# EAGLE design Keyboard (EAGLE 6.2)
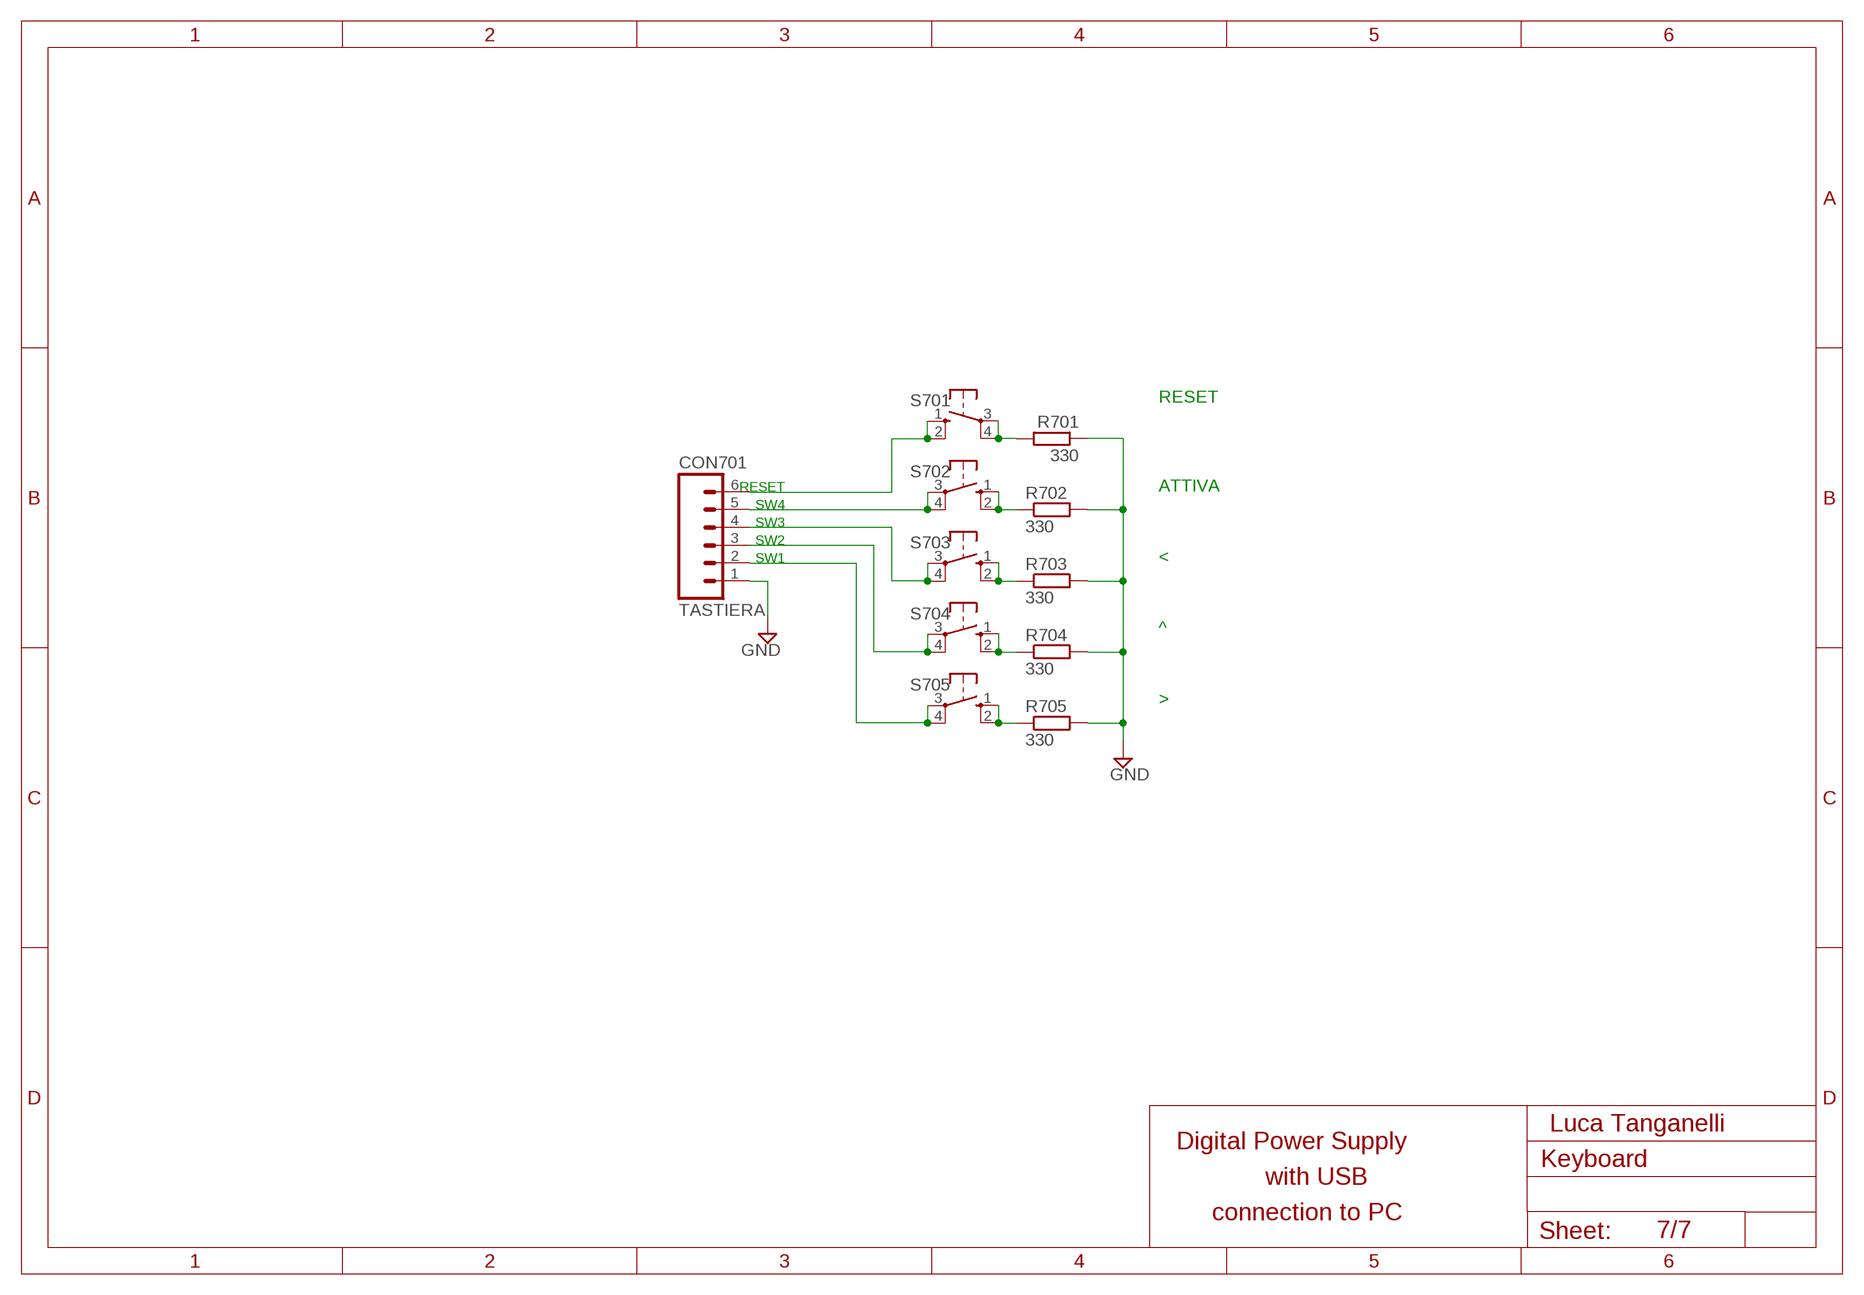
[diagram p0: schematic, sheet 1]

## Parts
CON701  TASTIERA  MA06  [06PA]
R701  330  R-EU_0207/10  [0207/10]
R702  330  R-EU_0207/10  [0207/10]
R703  330  R-EU_0207/10  [0207/10]
R704  330  R-EU_0207/10  [0207/10]
R705  330  R-EU_0207/10  [0207/10]
S701  10-XX  [B3F-10XX]
S702  10-XX  [B3F-10XX]
S703  10-XX  [B3F-10XX]
S704  10-XX  [B3F-10XX]
S705  10-XX  [B3F-10XX]

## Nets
GND: CON701.1 R701.1 R702.2 R703.2 R704.2 R705.2
N$1: CON701.5 S702.3(P) S702.4(P1)
N$2: CON701.4 S703.3(P) S703.4(P1)
N$3: CON701.3 S704.3(P) S704.4(P1)
N$4: CON701.2 S705.3(P) S705.4(P1)
N$10: R705.1 S705.1(S) S705.2(S1)
N$32: R701.2 S701.3(P) S701.4(P1)
N$86: R704.1 S704.1(S) S704.2(S1)
N$87: R703.1 S703.1(S) S703.2(S1)
N$88: R702.1 S702.1(S) S702.2(S1)
RESET1: CON701.6 S701.1(S) S701.2(S1)

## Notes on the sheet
- RESET
- RESET | ATTIVA
- SW4
- SW3
- SW2
- SW1 | <
- ^
- >
- Luca Tanganelli
- Digital Power Supply
- with USB
- connection to PC
- 7/7

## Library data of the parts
CON701 = #-con-amp-quick:MA06: AMP QUICK CONNECTOR; OC_FARNELL: unknown; OC_NEWARK: unknown
R701-R705 = #-rcl:R-EU_: RESISTOR, European symbol
S701-S705 = #-switch-omron:10-XX: OMRON SWITCH; MPN: B3F-1000; OC_FARNELL: 176432; OC_NEWARK: 36M3542

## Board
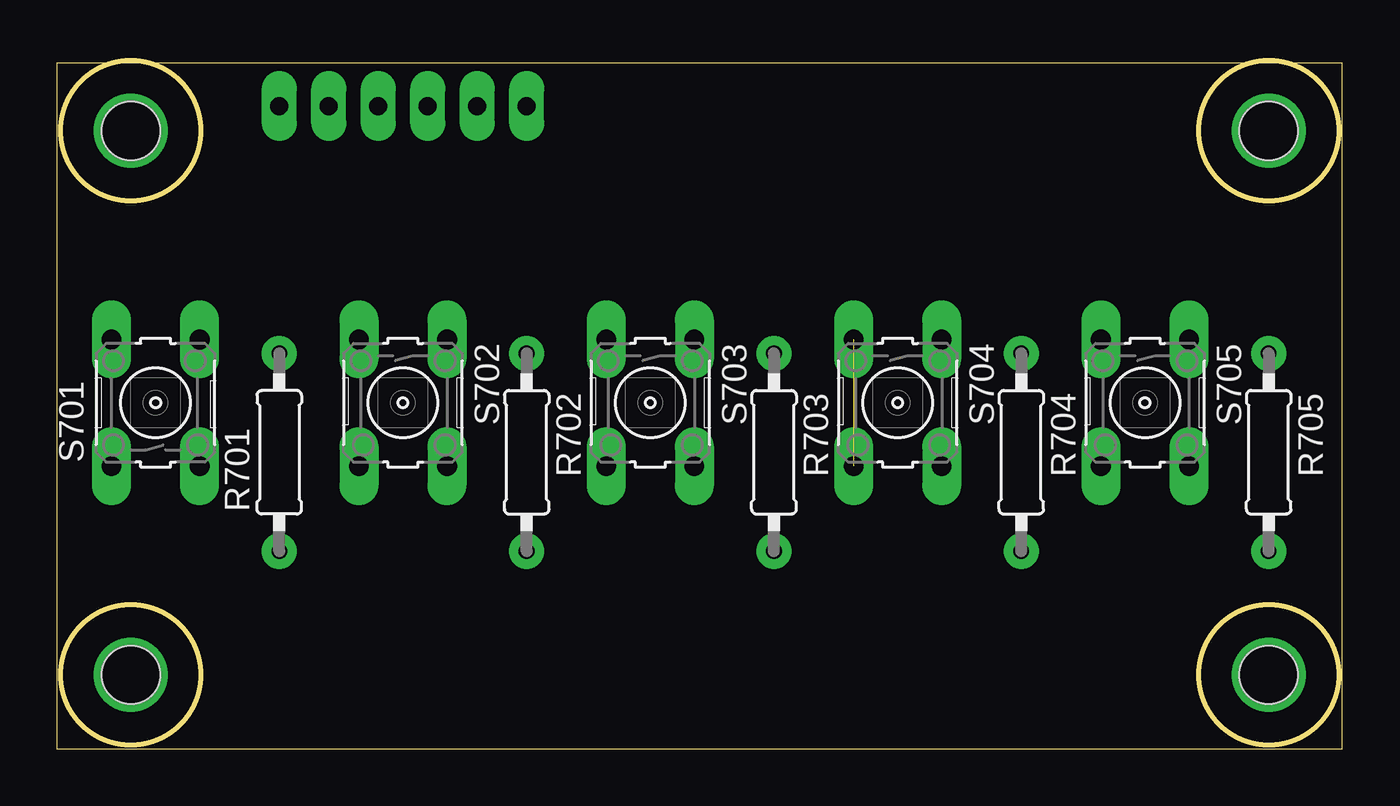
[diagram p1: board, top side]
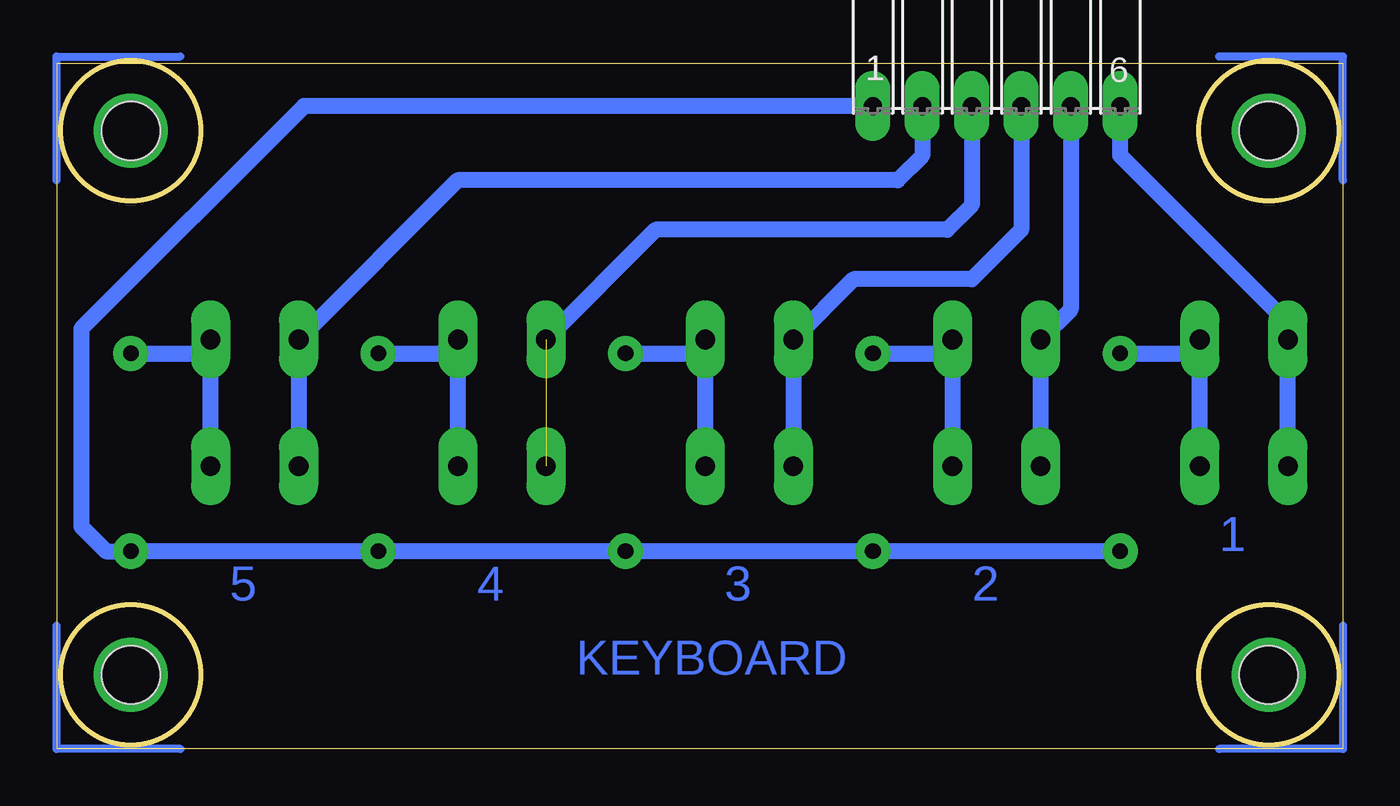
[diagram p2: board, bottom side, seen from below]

Size 66.02 x 35.34 mm. Coordinates in mm from the lower left corner, seen from the top.
Outline: 0,0 66.02,0 66.02,35.23 0,35.23 0,0
Outline: circle at 3.81,3.81 radius 3.59
Outline: circle at 3.81,31.75 radius 3.59
Outline: circle at 62.23,31.75 radius 3.59
Outline: circle at 62.23,3.81 radius 3.59
Copper layers (1*16): Top 0.035mm / dielectric 1.5mm / Bottom 0.035mm
Design rules: minimum track width 10mil, minimum drill 24mil, track to track 8mil, track to pad 8mil, pad to pad 8mil, via to via 8mil, smd to smd 8mil, copper to edge 40mil, drill to drill 8mil, minimum pad ring 10mil, minimum via ring 8mil, stop-mask expansion 4mil, vias tented up to drill 0mil, thermal gap 10mil
Holes 3 mm at 3.81,3.81 3.81,31.75 62.23,3.81 62.23,31.75

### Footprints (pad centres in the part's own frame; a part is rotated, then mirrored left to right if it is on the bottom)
06PA = drill 0.914 pad 1.8 long: 1 -6.35,0; 2 -3.81,0; 3 -1.27,0; 4 1.27,0; 5 3.81,0; 6 6.35,0
0207/10 = drill 0.8 pad 1.8: 1 -5.08,0; 2 5.08,0
B3F-10XX = drill 1.016 pad 2 long: 1 -3.251,2.261; 2 3.251,2.261; 3 -3.251,-2.261; 4 3.251,-2.261

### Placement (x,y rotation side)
CON701  17.78,33.02 0 bottom
R701  11.43,15.24 90 top
R702  24.13,15.24 270 top
R703  36.83,15.24 270 top
R704  49.53,15.24 270 top
R705  62.23,15.24 270 top
S701  5.08,17.78 90 top
S702  17.78,17.78 270 top
S703  30.48,17.78 270 top
S704  43.18,17.78 270 top
S705  55.88,17.78 270 top

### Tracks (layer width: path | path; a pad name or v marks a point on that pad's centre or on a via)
GND
  Bottom 0.813: R701.1 R702.2 R703.2 R704.2 R705.2 63.5,10.16 64.77,11.43 64.77,21.59 53.34,33.02 CON701.1
N$1
  Bottom 0.813: S702.4 S702.3 13.97,22.58 CON701.5
N$2
  Bottom 0.813: S703.4 S703.3 25.12,24.13 19.05,24.13 16.51,26.67 CON701.4
N$3  (1 unrouted)
  Bottom 0.813: CON701.3 19.05,27.94 20.32,26.67 35.28,26.67 S704.3
N$4
  Bottom 0.813: S705.4 S705.3 45.44,29.21 22.86,29.21 21.59,30.48 CON701.2
N$5  (via drill 1 pad 3.81)
  other vias: 3.81,3.81
N$6  (via drill 1 pad 3.81)
  other vias: 3.81,31.75
N$7  (via drill 1 pad 3.81)
  other vias: 62.23,3.81
N$8  (via drill 1 pad 3.81)
  other vias: 62.23,31.75
N$9
  Bottom 0.406: 0,6.35 0,0 6.35,0
N$10
  Bottom 0.813: S705.2 58.14,20.32 | 58.14,20.32 S705.1 | R705.1 58.14,20.32
N$11
  Bottom 0.406: 59.69,0 66.04,0 66.04,6.35
N$12
  Bottom 0.406: 66.04,29.21 66.04,35.56 59.69,35.56
N$13
  Bottom 0.406: 0,29.21 0,35.56 6.35,35.56
N$32
  Bottom 0.813: S701.3 7.34,20.32 | 7.34,20.32 S701.4 | R701.2 7.34,20.32
N$86
  Bottom 0.813: S704.1 45.44,20.32 | 45.44,20.32 S704.2 | R704.1 45.44,20.32
N$87
  Bottom 0.813: S703.1 32.74,20.32 | 32.74,20.32 S703.2 | R703.1 32.74,20.32
N$88
  Bottom 0.813: S702.1 20.04,20.32 | 20.04,20.32 S702.2 | R702.1 20.04,20.32
RESET1
  Bottom 0.813: S701.1 S701.2 2.82,21.87 11.43,30.48 CON701.6

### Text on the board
Bottom: 1 | 2 | 3 | 4 | 5 | KEYBOARD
